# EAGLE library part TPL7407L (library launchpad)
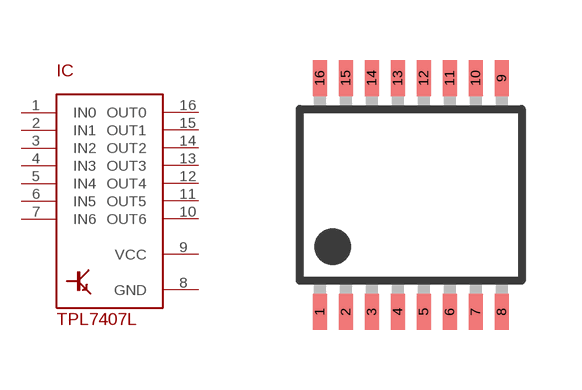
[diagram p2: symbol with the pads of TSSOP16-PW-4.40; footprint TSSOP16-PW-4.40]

Designator prefix IC

## TPL7407L  [TSSOP16-PW-4.40]
1  IN0
2  IN1
3  IN2
4  IN3
5  IN4
6  IN5
7  IN6
8  GND
9  VCC
10  OUT6
11  OUT5
12  OUT4
13  OUT3
14  OUT2
15  OUT1
16  OUT0

## Footprint TSSOP16-PW-4.40 (pad centres in mm)
smd 0.35 x 0.9: 1 -1.95,-2.925; 2 -1.3,-2.925; 3 -0.65,-2.925; 4 0,-2.925; 5 0.65,-2.925; 6 1.3,-2.925; 7 1.95,-2.925; 8 2.6,-2.925; 9 2.6,2.925; 10 1.95,2.925; 11 1.3,2.925; 12 0.65,2.925; 13 0,2.925; 14 -0.65,2.925; 15 -1.3,2.925; 16 -1.95,2.925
